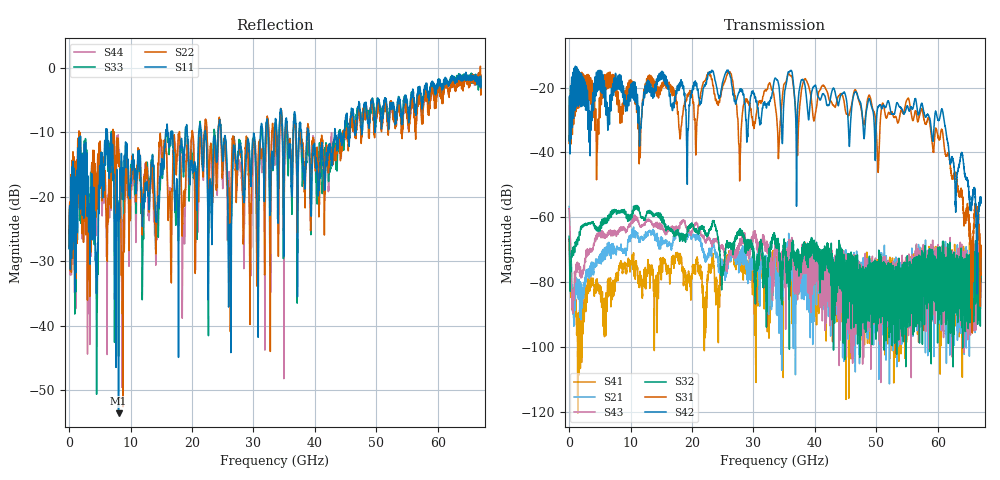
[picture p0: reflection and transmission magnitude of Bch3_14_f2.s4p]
!Agilent Technologies,N5247A,US51170199,A.09.90.13
!Agilent N5247A: A.09.90.13
!Date: Thursday, October 18, 2018 10:11:18
!Correction: S11(Full 4 Port(1,2,3,4))
!S12(Full 4 Port(1,2,3,4))
!S13(Full 4 Port(1,2,3,4))
!S14(Full 4 Port(1,2,3,4))
!S21(Full 4 Port(1,2,3,4))
!S22(Full 4 Port(1,2,3,4))
!S23(Full 4 Port(1,2,3,4))
!S24(Full 4 Port(1,2,3,4))
!S31(Full 4 Port(1,2,3,4))
!S32(Full 4 Port(1,2,3,4))
!S33(Full 4 Port(1,2,3,4))
!S34(Full 4 Port(1,2,3,4))
!S41(Full 4 Port(1,2,3,4))
!S42(Full 4 Port(1,2,3,4))
!S43(Full 4 Port(1,2,3,4))
!S44(Full 4 Port(1,2,3,4))
!S4P File: Measurements: <S11,S12,S13,S14>,
!<S21,S22,S23,S24>,
!<S31,S32,S33,S34>,
!<S41,S42,S43,S44>:
# Hz S  dB  R 50
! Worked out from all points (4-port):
!   6701 points, 10 MHz to 67 GHz, reference 50 ohm
!   strongest paths, dB at 10 MHz, 16.76 GHz, 33.51 GHz, 50.25 GHz, 67 GHz:
!     S42: -36.4, -26.5, -17.1, -26.1, -55.6
!     S31: -37.2, -21.4, -25.0, -44.8, -77.1
!     S32: -65.8, -64.4, -67.0, -81.7, -79.9
!     S43: -57.3, -62.8, -69.0, -80.3, -75.9
!     S21: -56.7, -68.5, -74.9, -77.0, -79.4
!     S41: -66.7, -73.1, -72.7, -85.6, -69.0
!   lowest |S11| = -53.6 dB at 8.049 GHz (marker M1), VSWR 1.00, Z = 49.8 + j0.0662 ohm
!   |S11| at or under -10 dB: start of sweep to 5.977 GHz; 6.226 GHz to 15.72 GHz (9.49 GHz wide, 86.5 % of centre); 24.73 GHz to 31.14 GHz (6.415 GHz wide, 23 % of centre)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
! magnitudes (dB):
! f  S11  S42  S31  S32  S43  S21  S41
! 10 MHz  -28.0  -36.4  -37.2  -65.8  -57.3  -56.7  -66.7
! 779.9 MHz  -19.0  -16.3  -20.7  -69.5  -84.1  -87.7  -85.1
! 8.049 GHz  -53.6  -18.1  -27.3  -58.0  -64.0  -69.4  -76.5
! 8.709 GHz  -15.8  -22.4  -25.2  -57.8  -63.4  -69.9  -77.0
! 26.16 GHz  -25.8  -16.0  -15.2  -68.0  -71.5  -72.2  -71.7
! 55.12 GHz  -6.3  -26.1  -23.3  -79.5  -72.0  -84.9  -89.2
! 67 GHz  -3.1  -55.6  -77.1  -79.9  -75.9  -79.4  -69.0
